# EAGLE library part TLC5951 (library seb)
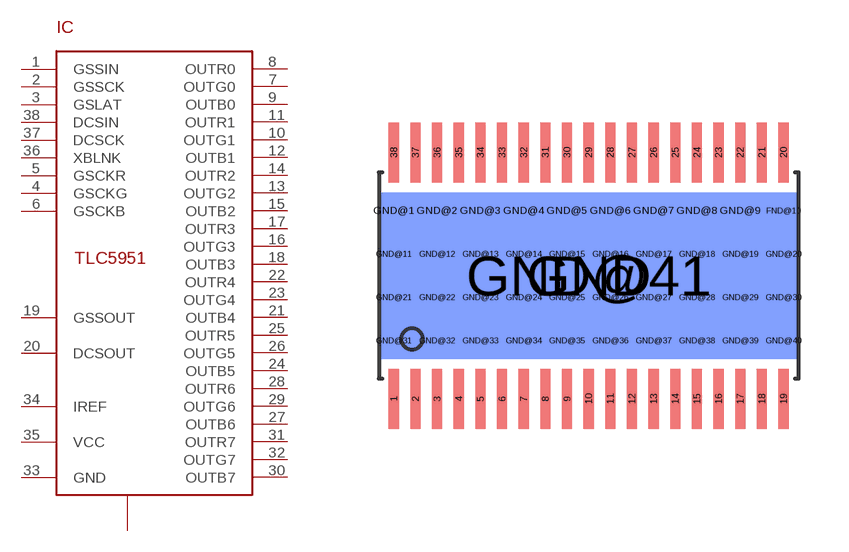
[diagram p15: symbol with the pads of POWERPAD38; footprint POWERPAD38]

Designator prefix IC

## TLC5951  [POWERPAD38]
1  GSSIN
2  GSSCK
3  GSLAT
4  GSCKG
5  GSCKR
6  GSCKB
7  OUTG0
8  OUTR0
9  OUTB0
10  OUTG1
11  OUTR1
12  OUTB1
13  OUTG2
14  OUTR2
15  OUTB2
16  OUTG3
17  OUTR3
18  OUTB3
19  GSSOUT
20  DCSOUT
21  OUTB4
22  OUTR4
23  OUTG4
24  OUTB5
25  OUTR5
26  OUTG5
27  OUTB6
28  OUTR6
29  OUTG6
30  OUTB7
31  OUTR7
32  OUTG7
33  GND
34  IREF
35  VCC
36  XBLNK
37  DCSCK
38  DCSIN
FND@10  GND
GND  GND
GND@1  GND
GND@2  GND
GND@3  GND
GND@4  GND
GND@5  GND
GND@6  GND
GND@7  GND
GND@8  GND
GND@9  GND
GND@11  GND
GND@12  GND
GND@13  GND
GND@14  GND
GND@15  GND
GND@16  GND
GND@17  GND
GND@18  GND
GND@19  GND
GND@20  GND
GND@21  GND
GND@22  GND
GND@23  GND
GND@24  GND
GND@25  GND
GND@26  GND
GND@27  GND
GND@28  GND
GND@29  GND
GND@30  GND
GND@31  GND
GND@32  GND
GND@33  GND
GND@34  GND
GND@35  GND
GND@36  GND
GND@37  GND
GND@38  GND
GND@39  GND
GND@40  GND
GND@41  GND

## Footprint POWERPAD38 (pad centres in mm)
smd 0.305 x 1.8: 1 -5.85,-3.7; 2 -5.2,-3.7; 3 -4.55,-3.7; 4 -3.9,-3.7; 5 -3.25,-3.7; 6 -2.6,-3.7; 7 -1.95,-3.7; 8 -1.3,-3.7; 9 -0.65,-3.7; 10 0,-3.7; 11 0.65,-3.7; 12 1.3,-3.7; 13 1.95,-3.7; 14 2.6,-3.7; 15 3.25,-3.7; 16 3.9,-3.7; 17 4.55,-3.7; 18 5.2,-3.7; 19 5.85,-3.7; 20 5.85,3.7; 21 5.2,3.7; 22 4.55,3.7; 23 3.9,3.7; 24 3.25,3.7; 25 2.6,3.7; 26 1.95,3.7; 27 1.3,3.7; 28 0.65,3.7; 29 0,3.7; 30 -0.65,3.7; 31 -1.3,3.7; 32 -1.95,3.7; 33 -2.6,3.7; 34 -3.25,3.7; 35 -3.9,3.7; 36 -4.55,3.7; 37 -5.2,3.7; 38 -5.85,3.7
drill 0.33 square: FND@10 5.85,1.95; GND@1 -5.85,1.95; GND@2 -4.55,1.95; GND@3 -3.25,1.95; GND@4 -1.95,1.95; GND@5 -0.65,1.95; GND@6 0.65,1.95; GND@7 1.95,1.95; GND@8 3.25,1.95; GND@9 4.55,1.95; GND@11 -5.85,0.65; GND@12 -4.55,0.65; GND@13 -3.25,0.65; GND@14 -1.95,0.65; GND@15 -0.65,0.65; GND@16 0.65,0.65; GND@17 1.95,0.65; GND@18 3.25,0.65; GND@19 4.55,0.65; GND@20 5.85,0.65; GND@21 -5.85,-0.65; GND@22 -4.55,-0.65; GND@23 -3.25,-0.65; GND@24 -1.95,-0.65; GND@25 -0.65,-0.65; GND@26 0.65,-0.65; GND@27 1.95,-0.65; GND@28 3.25,-0.65; GND@29 4.55,-0.65; GND@30 5.85,-0.65; GND@31 -5.85,-1.95; GND@32 -4.55,-1.95; GND@33 -3.25,-1.95; GND@34 -1.95,-1.95; GND@35 -0.65,-1.95; GND@36 0.65,-1.95; GND@37 1.95,-1.95; GND@38 3.25,-1.95; GND@39 4.55,-1.95; GND@40 5.85,-1.95
smd 12.5 x 5: GND 0,0
smd 12.5 x 5 bottom: GND@41 0,0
